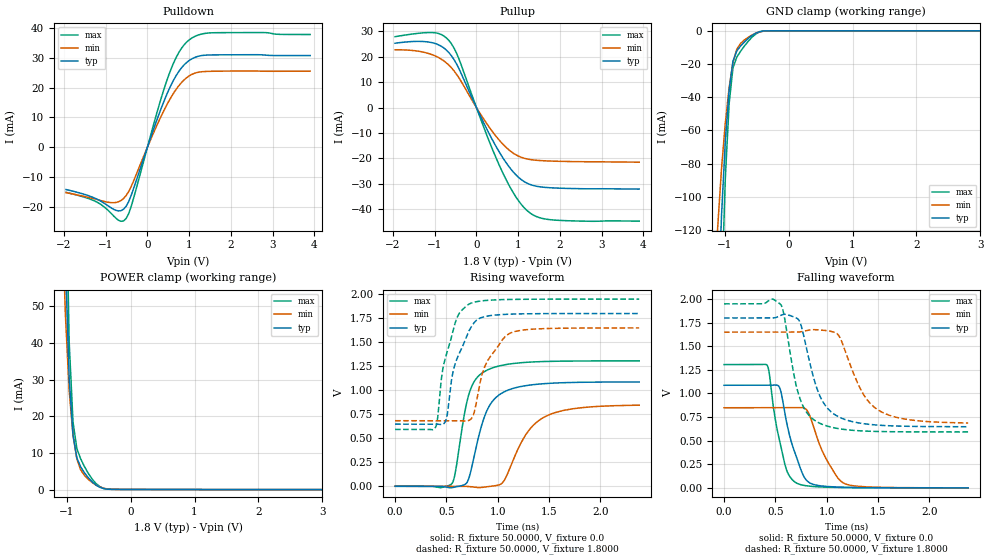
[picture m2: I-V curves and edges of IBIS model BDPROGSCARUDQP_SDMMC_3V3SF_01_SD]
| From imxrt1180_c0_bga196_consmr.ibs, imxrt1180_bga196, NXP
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[Model]  BDPROGSCARUDQP_SDMMC_3V3SF_01_SD
|   Model BDPROGSCARUDQP_SDMMC_3V3SF_01_SD
| This model was characterised for following simulation conditions:
| External (pad) voltage:
|   - Typ: 1.8V,   - Min: 1.65V,   - Max: 1.95V
| Library cells for typ/min/max conditions are connected as defined below:
|  IO - External Pad
|  A - Core Input
|  EN - Output Buffer Enable
|  ASRCN3V3[0] - gnde REFH3V3 gnde
|  ASRCN3V3[1] - REFH3V3 gnde gnde
|  ASRCN3V3[2] - gnde
|  ASRCN3V3[3] - gnde REFH3V3 gnde
|  ASRCP3V3[0] - vdde3v3 vdde3v3 REFL3V3
|  ASRCP3V3[1] - vdde3v3 REFL3V3 vdde3v3
|  ASRCP3V3[2] - REFL3V3 vdde3v3 vdde3v3
|  ASRCP3V3[3] - vdde3v3 REFL3V3 vdde3v3
|  IOGC - NC
|  PDRV - vdd
|  PSW - gnd
|  REFH3V3 - REFH3V3
|  REFL3V3 - REFL3V3
|  ZI - NC
|  gnd - gnd
|  gnde - gnde
|  vdd - vdd
|  vdde3v3 - vdde3v3
| All other pins connected to ground
Model_type I/O
Polarity   Non-Inverting
Enable   Active-Low
Vinl =   0.5800V
Vinh =   1.2700V
Vmeas =  0.9000V
Cref =   30.0000pF
Rref =   1.0000M
Vref =   1.8000V
C_comp   2.2202pF   2.2061pF   2.2431pF
|C_comp_pullup   1.1648pF   1.1334pF   1.1989pF
|C_comp_pulldown   0.7687pF   0.7946pF   0.7484pF
[Model Spec]
| variable   typ   min   max
Vinh   1.1700V   1.0725V   1.2675V
Vinl   0.6300V   0.5775V   0.6825V
[Temperature Range]   25.0000   0.1050k   -20.0000
[Voltage Range]   1.8000V   1.6500V   1.9500V
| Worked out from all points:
|   slope of the pulldown table from 0 to 0.27 V, typ, clamps not added: 24.9 ohm
|   slope of the pullup table from 0 to 0.27 V, typ, clamps not added: 29.4 ohm
|   GND clamp passes 1 mA (typ) near -0.49 V on its own axis
|   POWER clamp passes 1 mA (typ) near -0.52 V on its own axis
|   rising waveform, R_fixture 50.0000, V_fixture 0.0: 20-80 % time 187ps typ, 278ps min, 143ps max; typ from 0 V to 1.09 V
|   rising waveform, R_fixture 50.0000, V_fixture 1.8000: 20-80 % time 176ps typ, 209ps min, 151ps max; typ from 0.647 V to 1.8 V
|   falling waveform, R_fixture 50.0000, V_fixture 0.0: 20-80 % time 160ps typ, 207ps min, 131ps max; typ from 1.09 V to 0 V
|   falling waveform, R_fixture 50.0000, V_fixture 1.8000: 20-80 % time 199ps typ, 260ps min, 163ps max; typ from 1.8 V to 0.648 V
[Pulldown]
|Voltage   I(typ)   I(min)   I(max)
-1.95V    -14.21mA   -15.24mA   -15.16mA
-1.23V    -17.29mA   -17.49mA   -18.29mA
-870mV    -20.35mA   -18.61mA   -22.21mA
-630mV    -21.29mA   -17.87mA   -24.88mA
-510mV    -19.83mA   -16.21mA   -23.94mA
-390mV    -16.22mA   -13.24mA   -19.93mA
210mV     8.519mA    6.826mA    10.73mA
510mV     19.18mA    15.4mA     24.16mA
750mV     25.39mA    20.6mA     31.74mA
1.05V     29.56mA    24.36mA    36.54mA
1.59V     31mA       25.51mA    38.44mA
3.9V      30.78mA    25.54mA    37.85mA
[Pullup]
|Voltage   I(typ)   I(min)   I(max)
-1.95V    25.33mA    22.73mA    27.91mA
-1.38V    26.06mA    22.15mA    29.26mA
-960mV    25.07mA    20.12mA    29.37mA
-780mV    23.45mA    18.36mA    28.17mA
-600mV    20.41mA    15.67mA    25.13mA
-420mV    15.32mA    11.72mA    19.18mA
180mV     -6.218mA   -4.683mA   -7.944mA
600mV     -18.93mA   -13.83mA   -24.61mA
960mV     -26.73mA   -18.74mA   -35.55mA
1.26V     -30.13mA   -20.39mA   -41.21mA
1.86V     -31.66mA   -21.11mA   -44.29mA
3.9V      -32.11mA   -21.5mA    -44.72mA
[GND_clamp]
|Voltage   I(typ)   I(min)   I(max)
-1.95V    -1.789A    -1.03A     -2.95A
-1.11V    -176.3mA   -119.2mA   -277.9mA
-1.05V    -112.3mA   -83.66mA   -163.2mA
-990mV    -66.82mA   -55.78mA   -89.16mA
-930mV    -35.58mA   -34.18mA   -43.87mA
-870mV    -18.33mA   -19.06mA   -22.3mA
-810mV    -12.12mA   -11.08mA   -15.87mA
-750mV    -9.12mA    -7.575mA   -12.28mA
-570mV    -2.717mA   -2.477mA   -3.751mA
-450mV    -466.5uA   -625uA     -610.9uA
-330mV    -31.46uA   -57.07uA   -36.76uA
3.9V      0A         0A         0A
[POWER_clamp]
|Voltage   I(typ)   I(min)   I(max)
-1.95V    1.733A     983.2mA    2.899A
-1.08V    123mA      81.32mA    204.7mA
-1.02V    63.28mA    48.12mA    95.46mA
-960mV    30.45mA    27.05mA    40.34mA
-900mV    14.89mA    14.83mA    18.42mA
-840mV    8.668mA    8.37mA     11.21mA
-780mV    6.192mA    5.372mA    8.379mA
-720mV    4.573mA    3.84mA     6.25mA
-600mV    2.107mA    1.918mA    2.859mA
-480mV    625.6uA    714.7uA    800.1uA
-300mV    67.29uA    79.42uA    85.49uA
3.9V      0A         0A         0A
[Ramp]
| variable   typ   min   max
dV/dt_r  0.6518/0.1871n   0.5067/0.2778n   0.7834/0.1433n
dV/dt_f  0.6910/0.1987n   0.5773/0.2598n   0.8140/0.1626n
R_load = 50.0000
[Rising Waveform]
R_fixture= 50.0000
V_fixture= 0.0
V_fixture_min= 0.0
V_fixture_max= 0.0
|time   V(typ)   V(min)   V(max)
0s        166.1uV    140.5uV    208.2uV
551.8ps   -15.45mV   125uV      25.17mV
588.8ps   -5.716mV   208uV      150.4mV
669.4ps   13.92mV    477.8uV    711.8mV
719ps     82.64mV    -2.741mV   957.1mV
887.5ps   769.3mV    -6.272mV   1.205V
1.048ns   974.4mV    38.32mV    1.261V
1.275ns   1.048V     538.1mV    1.291V
1.464ns   1.07V      726.2mV    1.3V
2.38ns    1.087V     844.6mV    1.306V
[Rising Waveform]
R_fixture= 50.0000
V_fixture= 1.8000
V_fixture_min= 1.6500
V_fixture_max= 1.9500
|time   V(typ)   V(min)   V(max)
0s        647.2mV    682.9mV    592.2mV
393.6ps   647.6mV    683mV      612.8mV
485.6ps   665mV      683.1mV    1.317V
508.9ps   745.6mV    683.1mV    1.403V
573.7ps   1.229V     683.4mV    1.655V
724.3ps   1.625V     688.1mV    1.899V
768.7ps   1.7V       759.1mV    1.916V
880.3ps   1.768V     1.261V     1.935V
1.103ns   1.792V     1.583V     1.945V
2.38ns    1.799V     1.649V     1.949V
[Falling Waveform]
R_fixture= 50.0000
V_fixture= 0.0
V_fixture_min= 0.0
V_fixture_max= 0.0
|time   V(typ)   V(min)   V(max)
0s        1.087V     848.5mV    1.306V
421.4ps   1.086V     848.6mV    1.296V
533.7ps   1.076V     848.6mV    535.5mV
589.3ps   810.4mV    848.4mV    264.3mV
706.5ps   324mV      849.4mV    50.66mV
773.3ps   130.1mV    848.1mV    27.28mV
836.9ps   51.51mV    760.3mV    17.68mV
992ps     15.88mV    312.7mV    7.454mV
1.182ns   6.105mV    42.07mV    3.027mV
2.38ns    194.4uV    401.9uV    215.4uV
[Falling Waveform]
R_fixture= 50.0000
V_fixture= 1.8000
V_fixture_min= 1.6500
V_fixture_max= 1.9500
|time   V(typ)   V(min)   V(max)
0s        1.799V     1.649V     1.949V
550.9ps   1.826V     1.649V     1.943V
581ps     1.837V     1.649V     1.848V
724.9ps   1.783V     1.65V      994.8mV
796.4ps   1.512V     1.664V     812.7mV
919.6ps   1.01V      1.673V     691.4mV
1.117ns   751.8mV    1.615V     627.1mV
1.337ns   683.4mV    1.032V     603.4mV
1.497ns   664.7mV    828.2mV    597.2mV
2.38ns    647.5mV    687.1mV    592.3mV
